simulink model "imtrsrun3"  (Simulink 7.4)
settings: Solver=ode45  StartTime=0  StopTime=1.0  MaxStep=0.001  RelTol=1e-4  AbsTol=1e-4
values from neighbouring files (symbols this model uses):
  Hi = str2num(get(h,'string'))    [imic33.m]
  ic = [fs0 fr0]    [imdef0vec.m]    (also in imdef1vec.m; imdef2vec.m = F; imic2.m = [phids phiqs phidr phiqr n0]'; imic3.m = [phids phiqs phidr phiqr n0]')
  L = length(t)    [fourierdec.m]    (also in IMabc2.m = [Lss  Lsr; IMabcf0.m = [Lss  Lsr; IMabcf1.m = [Lss  Lsr; IMcur0.m = [Ls  0   Lm  0)
  Rr = input('Rotor resistance)[default = 2] =')    [Actac.m]    (also in im1phase.m = 0.3; im3d.m = eval(get(hRr,'String')); IMabc2.m = 0.02; imabcparam.m = 0.408)
  Rs = eval(get(hRs,'String'))    [im3d.m]    (also in IMabc2.m = 0.01; imabcparam.m = 0.531; IMabcrun0.m = 0.531; IMabcrun1.m = 0.531)
  Tl0 = Is*conj(Is)*Req    [imdef0vec.m]    (also in imdef1vec.m; imdef2vec.m = Lm*(I(2)*I(3)-I(1)*I(4)); imdefrotflux.m; imdefSIvec1.m = Te0/To)
  vs = 1.0    (= 1)    [imdef0vec.m]    (also in imdef1vec.m; imdef2vec.m; imdefrotflux.m; imdefSIvec1.m)
  wo = 2*pi*freq0    [calc0.m]    (also in IMabc2.m = 376.991118431; imabcparam.m = 376.991118431; IMabcrun0.m = 376.991118431; IMabcrun1.m = 376.991118431)
  ws = 1.0    (= 1)    [IMabc2.m]    (also in IMcur0.m; imdef0vec.m; imdef1vec.m; imdef2vec.m)
libraries: simulink x1

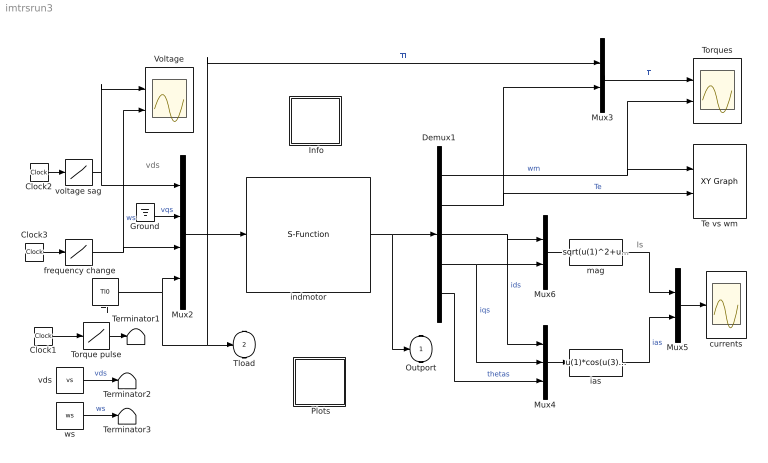
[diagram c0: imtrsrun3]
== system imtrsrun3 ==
  note: Is
  note: vds
  " Info" : Subsystem
  " Plots" : Subsystem
  " frequency change" : Lookup  InputValues=[0 0.1 0.1 0.5 0.5 2]  Table=[ws ws 0.8 0.8 ws ws]  OutDataType=sfix(16)  OutScaling=2^0
  Clock1 : Clock
  Clock2 : Clock
  Clock3 : Clock
  Demux1 : Demux  Outputs=5
  Ground : Ground
  Mux2 : Mux
  Mux3 : Mux  Inputs=2
  Mux4 : Mux  Inputs=3
  Mux5 : Mux  Inputs=2
  Mux6 : Mux  Inputs=2
  Te vs wm : simulink/Sinks/XY Graph  SystemSampleTime=-1  xmin=0.7  xmax=1  ymin=-3  ymax=4  st=0
  Terminator1 : Terminator
  Terminator2 : Terminator
  Terminator3 : Terminator
  Tl : Constant  Value=Tl0  OutDataType=sfix(16)  OutScaling=2^0
  Torque pulse : Lookup  InputValues=[0 0.1 0.1 0.5 0.5 2]  Table="[Tl0 Tl0  0 0 0.5 0.5]"  OutDataType=sfix(16)  OutScaling=2^0
  Torques : Scope  NumInputPorts=2
  Voltage : Scope  NumInputPorts=2
  currents : Scope
  ias : Fcn  Expr=u(1)*cos(u(3))-u(2)*sin(u(3))
  indmotor : S-Function  FunctionName=imKmoda  Parameters=Rs,Rr,L,Hi,wo,ic  EnableBusSupport=off
  mag : Fcn  Expr=sqrt(u(1)^2+u(2)^2)
  vds : Constant  Value=vs  OutDataType=sfix(16)  OutScaling=2^0
  voltage sag : Lookup  InputValues=[0 0.1 0.1 0.5 0.5 2]  Table="[vs vs  0.8 0.8 vs vs]"  OutDataType=sfix(16)  OutScaling=2^0
  ws : Constant  Value=ws  OutDataType=sfix(16)  OutScaling=2^0
  Outport : Outport
  Tload : Outport  Port=2
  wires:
  Mux4/1 -> ias/1
  Mux3/1 -> Torques/1  "T"
  Mux6/1 -> mag/1
  mag/1 -> Mux5/1
  ias/1 -> Mux5/2  "ias"
  Demux1/2 -> Te vs wm/2, Mux3/2  "Te"
  Demux1/5 -> Mux4/3  "thetas"
  Mux2/1 -> indmotor/1
  indmotor/1 -> Demux1/1, Outport/1
  Ground/1 -> Mux2/2  "vqs"
  Clock1/1 -> Torque pulse/1
  Torque pulse/1 -> Terminator1/1
  Tl/1 -> Mux2/4, Tload/1, Mux3/1  "Tl"
  Demux1/4 -> Mux6/2, Mux4/2  "iqs"
  Demux1/3 -> Mux6/1, Mux4/1  "ids"
  Demux1/1 -> Torques/2, Te vs wm/1  "wm"
  Mux5/1 -> currents/1
  ws/1 -> Terminator3/1  "ws"
  vds/1 -> Terminator2/1  "vds"
  Clock2/1 -> voltage sag/1
  Clock3/1 -> " frequency change"/1
  " frequency change"/1 -> Mux2/3, Voltage/2  "ws"
  voltage sag/1 -> Mux2/1, Voltage/1

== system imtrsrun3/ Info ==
  note: The induction machine is modeled here as an S-function. The demo simulates the running of an induction motor in steady-state when a sudden input change is effected: a)torque step changes at constant voltage excitation b) voltage input sag at constant frequency and load torque c)simultaneous step changes in voltage magnitude and frequency d) others
  note: Double click the block to enter the machine parameters and then establish the initial conditions

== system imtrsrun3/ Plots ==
  note: Plots
